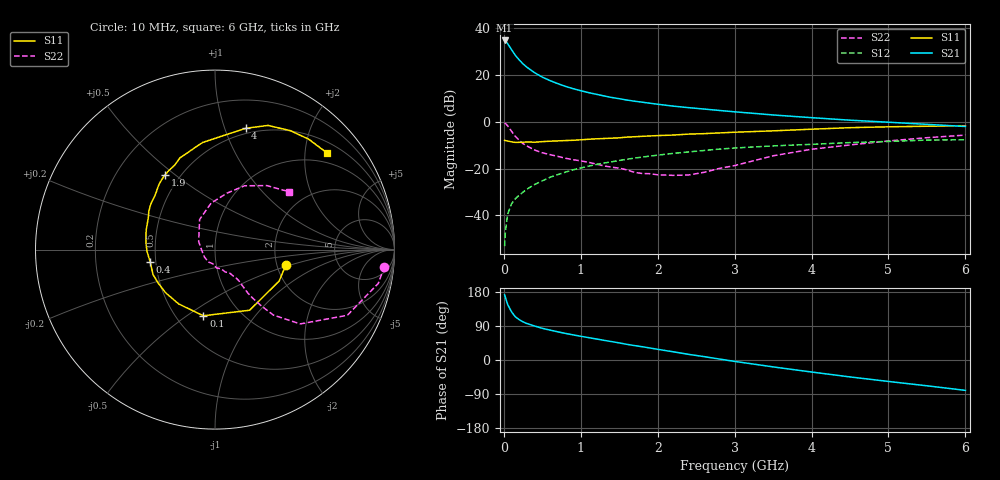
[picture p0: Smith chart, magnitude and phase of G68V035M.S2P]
! SIEMENS Small Signal Semiconductors
! BFG193
! Si NPN RF Bipolar Junction Transistor in SOT223
! VCE = 8 V  IC = 35 mA
! Common Emitter S-Parameters:  August  1996
# GHz  S  MA  R  50
!  f  S11  S21  S12  S22
! GHz  MAG  ANG  MAG  ANG  MAG  ANG  MAG  ANG
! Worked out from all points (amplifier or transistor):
!   36 points, 10 MHz to 6 GHz, reference 50 ohm
!   highest |S21| = 34.8 dB at 10 MHz (marker M1)
!   |S21| within 3 dB of that: start of sweep to 81.66 MHz
!   unconditionally stable (mu >= 1): 615.1 MHz to 2.45 GHz
!   at 250 MHz: K = 0.85, MSG = 27.4 dB, |S12| = -30.0 dB
!   at 1.4 GHz: K = 1.04, MAG = 12.5 dB, |S12| = -17.1 dB
!   at 6 GHz: K = 0.88, MSG = 2.8 dB, |S12| = -7.6 dB
!   S11 on the Smith chart (normalised r, x): 10 MHz: 2.23, -0.47; 100 MHz: 0.68, -0.58; 400 MHz: 0.47, -0.07; 1.9 GHz: 0.41, +0.46; 4 GHz: 0.45, +1.18; 6 GHz: 0.74, +2.48
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0.01  0.4037 -12.6  55.08 171.8  0.0022 89.5  0.9489 -5.7
0.02  0.3981 -26.1  53.63 165.4  0.0045 77.4  0.9291 -11.7
0.05  0.389 -60.3  46.94 146.4  0.0107 71.5  0.8231 -26.4
0.1  0.3743 -100.0  35.02 127.0  0.0177 66.1  0.6299 -41.1
0.15  0.3641 -123.8  26.45 113.9  0.0228 63.1  0.4885 -48.3
0.2  0.3655 -139.0  21.1 106.4  0.0271 64.1  0.4042 -50.6
0.25  0.3674 -149.5  17.36 100.6  0.0315 64.3  0.3421 -52.2
0.3  0.3723 -158.0  14.74 96.2  0.0365 65.3  0.3051 -52.9
0.4  0.3676 -169.6  11.27 89.7  0.0458 66.1  0.25 -52.8
0.5  0.3784 -178.0  9.062 83.6  0.0549 65.7  0.2184 -52.5
0.6  0.3862 174.8  7.636 78.9  0.0653 65.2  0.1997 -53.3
0.7  0.3919 169.0  6.582 74.4  0.0744 64.4  0.1831 -55.1
0.9  0.4039 159.1  5.138 66.3  0.0944 61.1  0.1555 -57.7
1.1  0.4245 150.4  4.228 59.1  0.1128 58.1  0.1368 -65.5
1.4  0.4479 138.9  3.329 48.6  0.14 52.0  0.1075 -78.0
1.9  0.5001 124.0  2.505 31.6  0.1857 41.6  0.078 -115.5
2.2  0.5225 115.3  2.175 21.7  0.2118 34.7  0.0719 -145.7
3.5  0.6431 84.5  1.406 -18.2  0.3065 4.0  0.1884 117.1
4  0.6971 75.8  1.23 -31.7  0.331 -5.7  0.2598 94.8
4.5  0.7522 66.9  1.087 -44.7  0.3612 -15.8  0.3211 78.1
5.5  0.8068 49.7  0.885 -68.1  0.4078 -38.9  0.4588 51.0
6  0.8237 41.0  0.797 -80.1  0.4148 -52.4  0.5222 38.2
